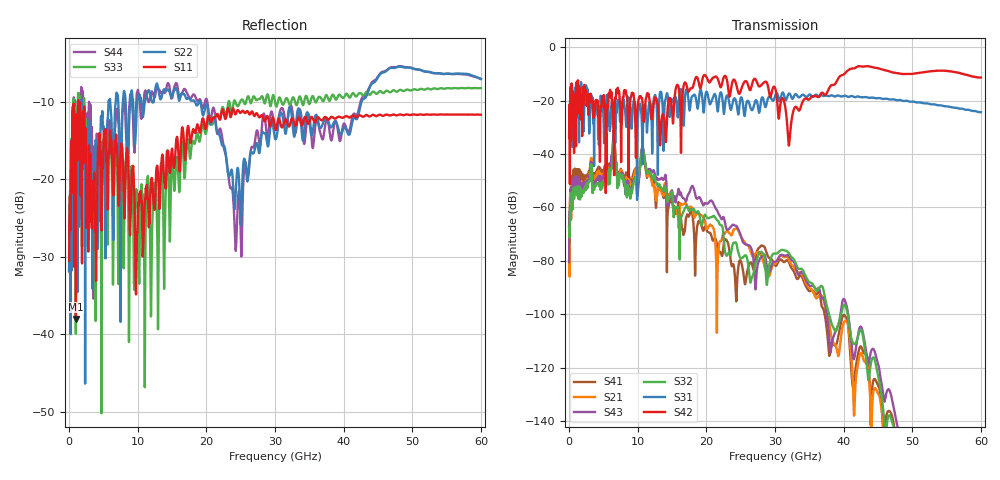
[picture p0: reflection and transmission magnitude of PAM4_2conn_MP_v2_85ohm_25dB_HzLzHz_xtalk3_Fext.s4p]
! Info: Touchstone file created by Circ.  Input file=FAB50GbE_2conn_Midplane_Examax_Topo2_v2_85ohm_25dB_HzLzHz.circ
# Hz S RI R 50
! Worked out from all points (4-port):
!   6000 points, 10 MHz to 60 GHz, reference 50 ohm
!   strongest paths, dB at 10 MHz, 15.01 GHz, 30.01 GHz, 45.01 GHz, 60 GHz:
!     S42: -34.0, -24.0, -15.3, -7.9, -11.4
!     S31: -33.9, -19.6, -18.3, -19.1, -24.4
!     S32: -67.5, -54.5, -77.3, -122.8, -168.2
!     S43: -80.5, -53.7, -80.4, -118.6, -175.5
!     S21: -63.7, -56.0, -81.0, -129.7, -173.5
!     S41: -66.9, -57.2, -81.7, -126.6, -190.2
!   lowest |S11| = -38.1 dB at 1 GHz (marker M1), VSWR 1.03, Z = 50.1 + j1.25 ohm
!   |S11| at or under -10 dB: start of sweep to 1.316 GHz; 1.357 GHz to end of sweep
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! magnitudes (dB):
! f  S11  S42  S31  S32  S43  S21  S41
! 10 MHz  -30.5  -34.0  -33.9  -67.5  -80.5  -63.7  -66.9
! 1 GHz  -38.1  -26.5  -18.1  -53.4  -50.5  -50.9  -48.0
! 10.76 GHz  -29.4  -23.4  -31.9  -38.2  -37.5  -38.7  -38.1
! 23.85 GHz  -10.9  -12.7  -20.5  -73.8  -66.5  -69.3  -81.5
! 32.06 GHz  -13.2  -36.5  -17.3  -77.3  -78.3  -79.7  -80.7
! 42.09 GHz  -11.9  -7.2  -18.4  -108.5  -107.9  -118.6  -115.1
! 60 GHz  -11.7  -11.4  -24.4  -168.2  -175.5  -173.5  -190.2
